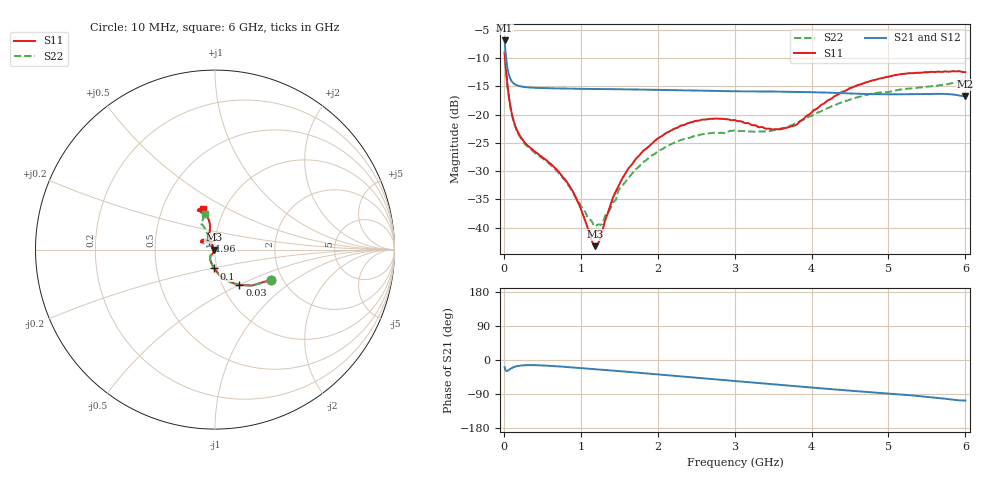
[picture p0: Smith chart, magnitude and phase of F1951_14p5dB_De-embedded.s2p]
! Integrated Device Technology
! Corporate Headquarters
! 6024 Silver Creek Valley Road
! San Jose, CA 95138  USA
! Phone:  1-408-284-8200
! Toll Free:  1-800-223-1366
! Webpage:  http://www.idt.com/
! Timing and RF Division
! 515 Groton Road, Suite 102
! Westford, MA 01886-6024
! Device:  F1951
! Description: 6-bit 0.5 dB Digital Step Attenuator
! Frequency:  100.0 -  4000.00 MHz
! Package:  4x4 mm Thin QFN Plastic Package: 24 pin
! Ports:  2 RF, 6 DC
!  Pin  1  = NC
!  Pin  2  = RF1  =  Port 1
!  Pin  3  = GND
!  Pin  4  = NC
!  Pin  5  = Serial Data Out (SDO)
!  Pin  6  = NC
!  Pin  7  = Reset Bar ( RSTb)
!  Pin  8  = Clock (CLK)
!  Pin  9  = Chip Select Bar (CSb)
!  Pin 10  = NC
!  Pin 11  = Serial Data In (SDI)
!  Pin 12  = NC
!  Pin 13  = NC
!  Pin 14  = VDD
!  Pin 15  = NC
!  Pin 16  = GND
!  Pin 17  = RF2  =  Port 2
!  Pin 18  = NC
!  Pin 19  = GND
!  Pin 20  = GND
!  Pin 21  = GND
!  Pin 22  = GND
!  Pin 23  = GND
!  Pin 24  = GND
! State:  29
! Atten State:  14.5 dB
! Voltage:  +3.30 Volts
! Current:  0.488 mA
! Data:  The device was measured on a F195X evaluation board which has
!  individual transmission lines to the RF pins.  Data was collected
!  de-embedded using a Automatic Fixture Removal [AFR] (Keysight Technologies).
!  The reference plane is the edge of the package pin.
! Misc:  Lot Code  1225BCA
!  Action Tracker AT0399
! Date Measured:  2018-09-13
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# GHz S dB R 50
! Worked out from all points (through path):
!   600 points, 10 MHz to 6 GHz, reference 50 ohm
!   highest |S21| = -6.86 dB at 10 MHz (marker M1); lowest = -16.8 dB at 6 GHz (marker M2)
!   group delay of S21, straight-line fit = 45.3 ps
!   lowest |S11| = -43.3 dB at 1.19 GHz (marker M3), VSWR 1.01, Z = 49.3 + j0.00757 ohm
!   |S11| at or under -10 dB: 15.62 MHz to end of sweep
!   |S22| runs from -39.8 to -9.0 dB; largest |S21 - S12| = 0.00035
!   S11 on the Smith chart (normalised r, x): 10 MHz: 1.75, -0.67; 30 MHz: 1.20, -0.50; 100 MHz: 0.97, -0.21; 1.96 GHz: 0.93, +0.09; 6 GHz: 0.80, +0.39
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0.01  -8.97 -28.0  -6.86 -18.9  -6.86 -18.9  -8.95 -28.5
0.03  -12.42 -55.3  -9.99 -28.8  -9.99 -28.9  -12.50 -56.1
0.06  -16.25 -76.7  -12.65 -27.1  -12.65 -27.1  -16.39 -77.6
0.1  -19.59 -92.2  -14.04 -21.6  -14.04 -21.6  -19.70 -93.4
0.17  -22.72 -107.6  -14.80 -16.3  -14.79 -16.3  -22.91 -108.9
0.26  -24.73 -117.4  -15.09 -13.9  -15.09 -13.9  -24.99 -119.3
0.72  -30.22 -122.1  -15.36 -16.9  -15.35 -17.0  -30.46 -129.1
0.88  -33.22 -122.2  -15.40 -19.3  -15.40 -19.4  -33.35 -130.9
1.01  -37.03 -126.8  -15.43 -21.3  -15.43 -21.3  -36.32 -136.2
1.19  -43.30 179.4  -15.45 -24.1  -15.45 -24.2  -39.83 -170.4
1.28  -40.69 138.1  -15.46 -25.7  -15.46 -25.7  -39.34 164.1
1.41  -35.04 120.0  -15.49 -27.9  -15.49 -27.9  -35.86 141.9
1.54  -31.29 117.7  -15.51 -30.0  -15.51 -30.0  -32.57 133.1
1.96  -24.69 125.7  -15.60 -37.5  -15.60 -37.5  -26.98 133.6
2.01  -24.15 127.4  -15.61 -38.4  -15.61 -38.4  -26.40 134.7
2.49  -21.10 141.2  -15.73 -46.8  -15.73 -46.8  -23.76 144.2
3.01  -20.99 151.7  -15.85 -55.7  -15.86 -55.7  -22.81 148.5
3.59  -22.61 130.8  -15.92 -65.6  -15.92 -65.6  -22.48 130.2
4.01  -19.47 105.9  -16.02 -72.9  -16.02 -72.8  -20.14 117.4
4.49  -15.36 102.0  -16.24 -80.8  -16.24 -80.8  -17.37 115.6
5.01  -13.24 109.7  -16.40 -88.5  -16.40 -88.4  -15.98 118.0
6  -12.47 105.7  -16.77 -107.1  -16.77 -107.1  -13.76 105.6
